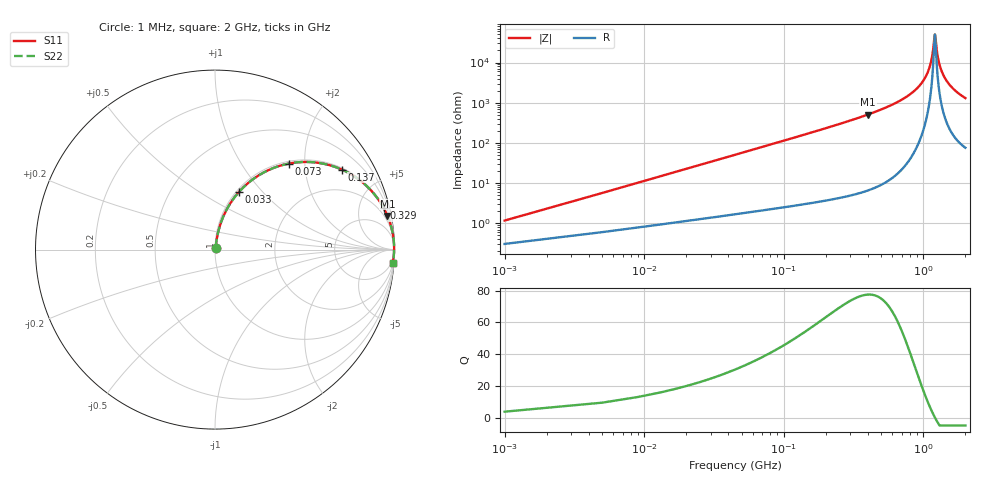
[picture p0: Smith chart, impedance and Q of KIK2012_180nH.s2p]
!version-2
!date-01.2022
!Series
# MHz S RI R 50
!Freq ReS11 ImS11 ReS21 ImS21 ReS12 ImS12 ReS22 ImS22
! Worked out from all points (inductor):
!   501 points, 1 MHz to 2 GHz, reference 50 ohm
!   read as one part in series: L = 180 nH near 9 MHz
!   highest Q = 77.5 at 401 MHz (marker M1), where L = 202 nH
!   self-resonance near 1.209 GHz
!   S11 on the Smith chart (normalised r, x): 1 MHz: 1.01, +0.02; 33 MHz: 1.03, +0.75; 73 MHz: 1.04, +1.66; 137 MHz: 1.06, +3.14; 329 MHz: 1.11, +8.04; 2 GHz: 3, -26
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1  0.00319 0.0112  0.9968 -0.0112  0.9968 -0.0112  0.00319 0.0112
13  0.0298 0.1413  0.9702 -0.1413  0.9702 -0.1413  0.0298 0.1413
21  0.0632 0.22  0.9368 -0.22  0.9368 -0.22  0.0632 0.22
33  0.1319 0.3196  0.8681 -0.3196  0.8681 -0.3196  0.1319 0.3196
73  0.4095 0.479  0.5905 -0.479  0.5905 -0.479  0.4095 0.479
137  0.7078 0.4455  0.2922 -0.4455  0.2922 -0.4455  0.7078 0.4455
213  0.857 0.3425  0.143 -0.3425  0.143 -0.3425  0.857 0.3425
329  0.939 0.2329  0.061 -0.2329  0.061 -0.2329  0.939 0.2329
337  0.942 0.2272  0.058 -0.2272  0.058 -0.2272  0.942 0.2272
401  0.9607 0.188  0.0393 -0.188  0.0393 -0.188  0.9607 0.188
669  0.9901 0.0907  0.00987 -0.0907  0.00987 -0.0907  0.9901 0.0907
1001  0.9976 0.0278  0.00243 -0.0278  0.00243 -0.0278  0.9976 0.0278
1073  0.9979 0.0175  0.00206 -0.0175  0.00206 -0.0175  0.9979 0.0175
1129  0.9981 0.0101  0.00195 -0.0101  0.00195 -0.0101  0.9981 0.0101
1165  0.9981 0.00551  0.00194 -0.00551  0.00194 -0.00551  0.9981 0.00551
1209  0.998 0.000117  0.00199 -0.000117  0.00199 -0.000117  0.998 0.000117
1217  0.998 -0.000842  0.00201 0.000842  0.00201 0.000842  0.998 -0.000842
1269  0.9978 -0.00693  0.00217 0.00693  0.00217 0.00693  0.9978 -0.00693
1337  0.9975 -0.0145  0.00249 0.0145  0.00249 0.0145  0.9975 -0.0145
1469  0.9966 -0.0283  0.00342 0.0283  0.00342 0.0283  0.9966 -0.0283
1669  0.9945 -0.0474  0.00548 0.0474  0.00548 0.0474  0.9945 -0.0474
2000  0.9898 -0.0754  0.0102 0.0754  0.0102 0.0754  0.9898 -0.0754
